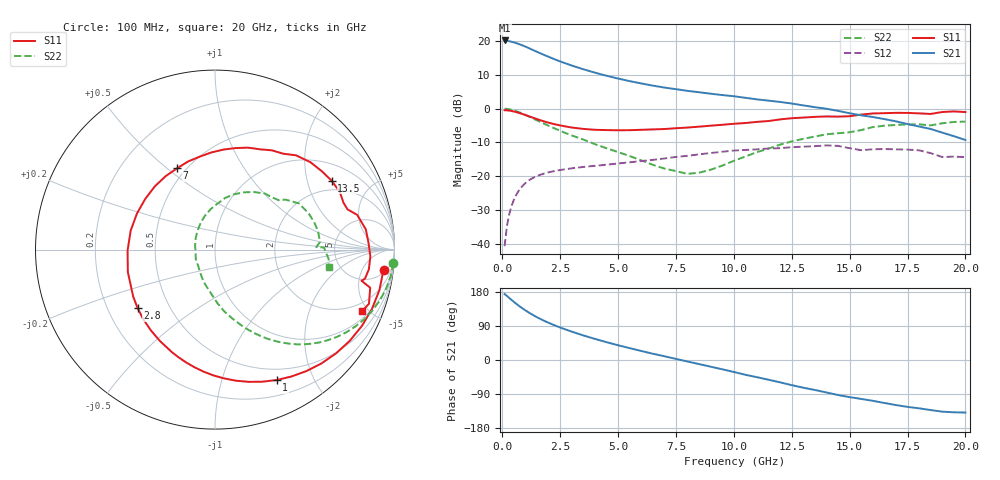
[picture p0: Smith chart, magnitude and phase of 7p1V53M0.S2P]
! Infineon Technologies  Discrete & RF Semiconductors
! bfp620
! VCE =  1.5 V,  IC =  3.0 mA
! Common Emitter S-Parameters:  Sep 2002
# GHz  S  MA  R  50
!  f  S11  S21  S12  S22
! GHz  MAG  ANG  MAG  ANG  MAG  ANG  MAG  ANG
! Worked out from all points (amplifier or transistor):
!   59 points, 100 MHz to 20 GHz, reference 50 ohm
!   highest |S21| = 20.1 dB at 100 MHz (marker M1)
!   |S21| within 3 dB of that: start of sweep to 1.382 GHz
!   unconditionally stable (mu >= 1): 5.403 GHz to 12.32 GHz; 14.38 GHz to 15.6 GHz; 17.25 GHz to end of sweep
!   at 1 GHz: K = 0.21, MSG = 20.1 dB, |S12| = -22.0 dB
!   at 5.5 GHz: K = 1.01, MAG = 11.4 dB, |S12| = -15.9 dB
!   at 20 GHz: K = 1.43, MAG = -1.4 dB, |S12| = -14.3 dB
!   S11 on the Smith chart (normalised r, x): 100 MHz: 6, -14; 1 GHz: 0.37, -1.52; 2.8 GHz: 0.33, -0.30; 7 GHz: 0.45, +0.54; 13.5 GHz: 1.59, +2.84; 20 GHz: 1.42, -4.61
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0.1  0.9458 -6.8  10.15 174.1  0.0093 84.5  0.9969 -4.4
0.3  0.9351 -20.7  9.88 163.7  0.0276 79.0  0.9777 -13.0
0.5  0.9066 -34.1  9.503 153.4  0.0451 71.4  0.9404 -21.2
0.6  0.8883 -40.6  9.28 148.5  0.0531 67.7  0.9171 -25.1
0.8  0.8472 -53.0  8.778 139.3  0.0675 60.7  0.8645 -32.2
1  0.8036 -64.7  8.227 130.9  0.0795 54.5  0.8077 -38.6
1.2  0.7604 -75.7  7.67 123.2  0.0895 48.9  0.7505 -44.3
1.4  0.7197 -85.9  7.142 116.1  0.0977 44.1  0.696 -49.3
1.8  0.6487 -104.4  6.223 103.7  0.1098 36.3  0.5999 -57.5
2.2  0.5945 -121.1  5.457 93.0  0.1186 30.4  0.521 -64.2
2.8  0.5399 -143.1  4.577 79.2  0.1284 23.6  0.4263 -72.7
3.5  0.5015 -165.5  3.815 64.8  0.1377 17.4  0.3491 -81.4
4  0.487 -179.5  3.395 55.7  0.1429 13.7  0.2988 -87.4
5  0.4791 155.0  2.781 38.9  0.1548 7.9  0.2282 -98.6
6  0.4864 133.6  2.356 23.8  0.1679 2.4  0.1721 -115.0
7  0.4997 115.1  2.047 9.9  0.1834 -2.9  0.1301 -136.1
8.5  0.5415 92.2  1.745 -10.8  0.2112 -13.0  0.1132 169.0
10.5  0.6126 65.8  1.444 -39.0  0.2455 -30.9  0.1965 106.6
12  0.6928 49.3  1.254 -59.0  0.2606 -43.5  0.2939 78.8
13.5  0.7549 30.6  1.05 -79.1  0.2791 -58.1  0.3871 56.0
17  0.8663 -2.5  0.649 -118.9  0.2504 -88.9  0.5734 15.3
20  0.8894 -22.5  0.344 -138.7  0.1924 -106.6  0.6427 -8.6
